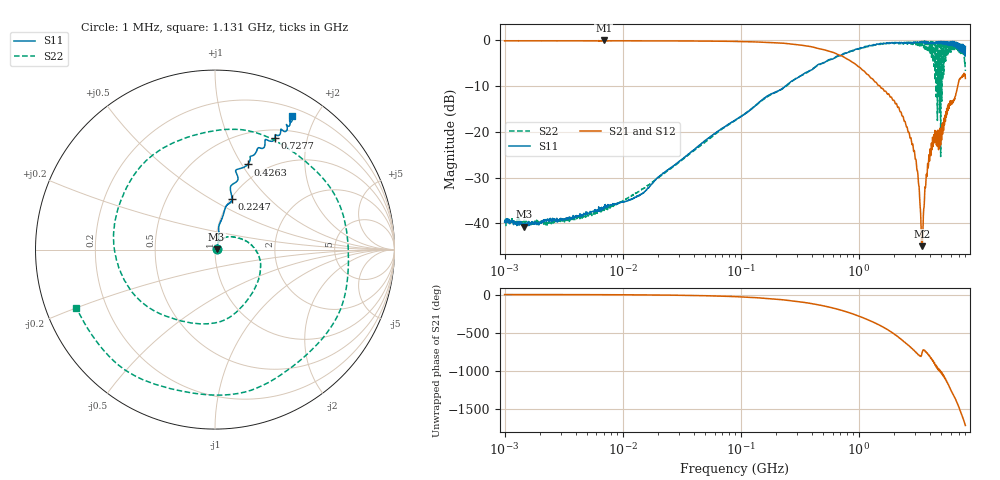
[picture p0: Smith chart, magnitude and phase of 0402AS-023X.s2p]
!s-Parameter Generated by FASTRON Sdn. Bhd.
!FASTRON P/N : 0402AS-023X
!Keysight Technologies: E5071C_MY46733604_B.14.02
!Date: Mon Dec 01 10:33:14 2025
!Version  :Rev00  Mon Dec 01 10:33:14 2025
!Data & Calibration Information:
!Freq  S11:SOLT2(ON)  S21:SOLT2(ON)  S12:SOLT2(ON)  S22:SOLT2(ON)
!PortZ  Port1:50+j0  Port2:50+j0
!When reading reference impedance value at option line is always used.
! Remarks : This data is being provided solely for informational purposes.
# Hz S dB R 50
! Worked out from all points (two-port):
!   1601 points, 1 MHz to 8 GHz, reference 50 ohm
!   highest |S21| = -0.02 dB at 6.912 MHz (marker M1); lowest = -45.0 dB at 3.426 GHz (marker M2)
!   |S21| within 3 dB of the highest: start of sweep to 655.4 MHz
!   lowest |S11| = -40.7 dB at 1.459 MHz (marker M3), VSWR 1.02, Z = 50.9 + j0.202 ohm
!   |S11| at or under -10 dB: start of sweep to 238.1 MHz
!   |S22| runs from -40.5 to -0.1 dB; largest |S21 - S12| = 0.018
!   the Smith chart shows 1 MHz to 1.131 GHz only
!   S11 on the Smith chart (normalised r, x): 1 MHz: 1.02, +0.00; 224.7 MHz: 1.01, +0.63; 426.3 MHz: 0.83, +1.06; 727.7 MHz: 0.61, +1.50; 1.131 GHz: 0.30, +1.69
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1000000  -39.70 13.4  -0.10 -0.3  -0.09 -0.3  -39.20 10.0
1459186  -40.70 12.4  -0.08 -0.5  -0.08 -0.5  -39.60 5.0
4479405  -38.10 32.2  -0.10 -1.5  -0.09 -1.5  -38.90 34.1
6911657  -36.40 36.1  -0.02 -2.7  -0.13 -2.0  -36.40 37.3
2.00676e7  -29.90 63.0  -0.11 -6.4  -0.11 -6.3  -30.00 61.8
8.994653e7  -17.40 80.5  -0.23 -27.9  -0.22 -27.8  -17.50 30.8
2.247047e8  -10.50 71.4  -0.61 -68.3  -0.60 -68.3  -10.60 -35.1
4.006501e8  -6.45 72.2  -1.41 -120.0  -1.40 -120.0  -6.31 -136.0
4.262922e8  -5.87 68.9  -1.59 -128.0  -1.58 -128.0  -5.85 -148.0
7.276733e8  -3.03 61.7  -3.48 148.0  -3.47 148.0  -3.15 53.1
1.131415e9  -1.32 60.2  -6.93 42.9  -6.93 42.8  -1.53 -157.0
1.349549e9  -0.96 63.5  -8.90 -9.0  -8.92 -9.1  -1.00 95.0
1.542898e9  -0.70 68.2  -10.40 -53.5  -10.40 -53.6  -0.76 1.2
1.7949e9  -0.56 73.9  -11.80 -112.0  -11.80 -112.0  -0.72 -121.0
2.082516e9  -0.53 80.0  -13.80 180.0  -13.80 180.0  -0.71 96.4
2.44288e9  -0.64 84.9  -17.70 95.4  -17.70 95.3  -0.44 -78.2
2.809687e9  -0.49 94.8  -22.60 12.7  -22.60 12.5  -0.45 101.0
3.183204e9  -0.39 104.0  -30.20 -71.4  -30.20 -71.7  -0.74 -88.0
3.42643e9  -0.46 109.0  -45.00 -53.7  -45.00 -52.6  -0.61 163.0
3.730463e9  -0.62 116.0  -29.30 -37.4  -29.30 -37.9  -1.22 13.5
4.115571e9  -0.70 125.0  -22.50 -119.0  -22.50 -119.0  -1.17 -164.0
8e9  -1.33 -105.0  -8.32 78.4  -8.35 77.9  -6.70 132.0
